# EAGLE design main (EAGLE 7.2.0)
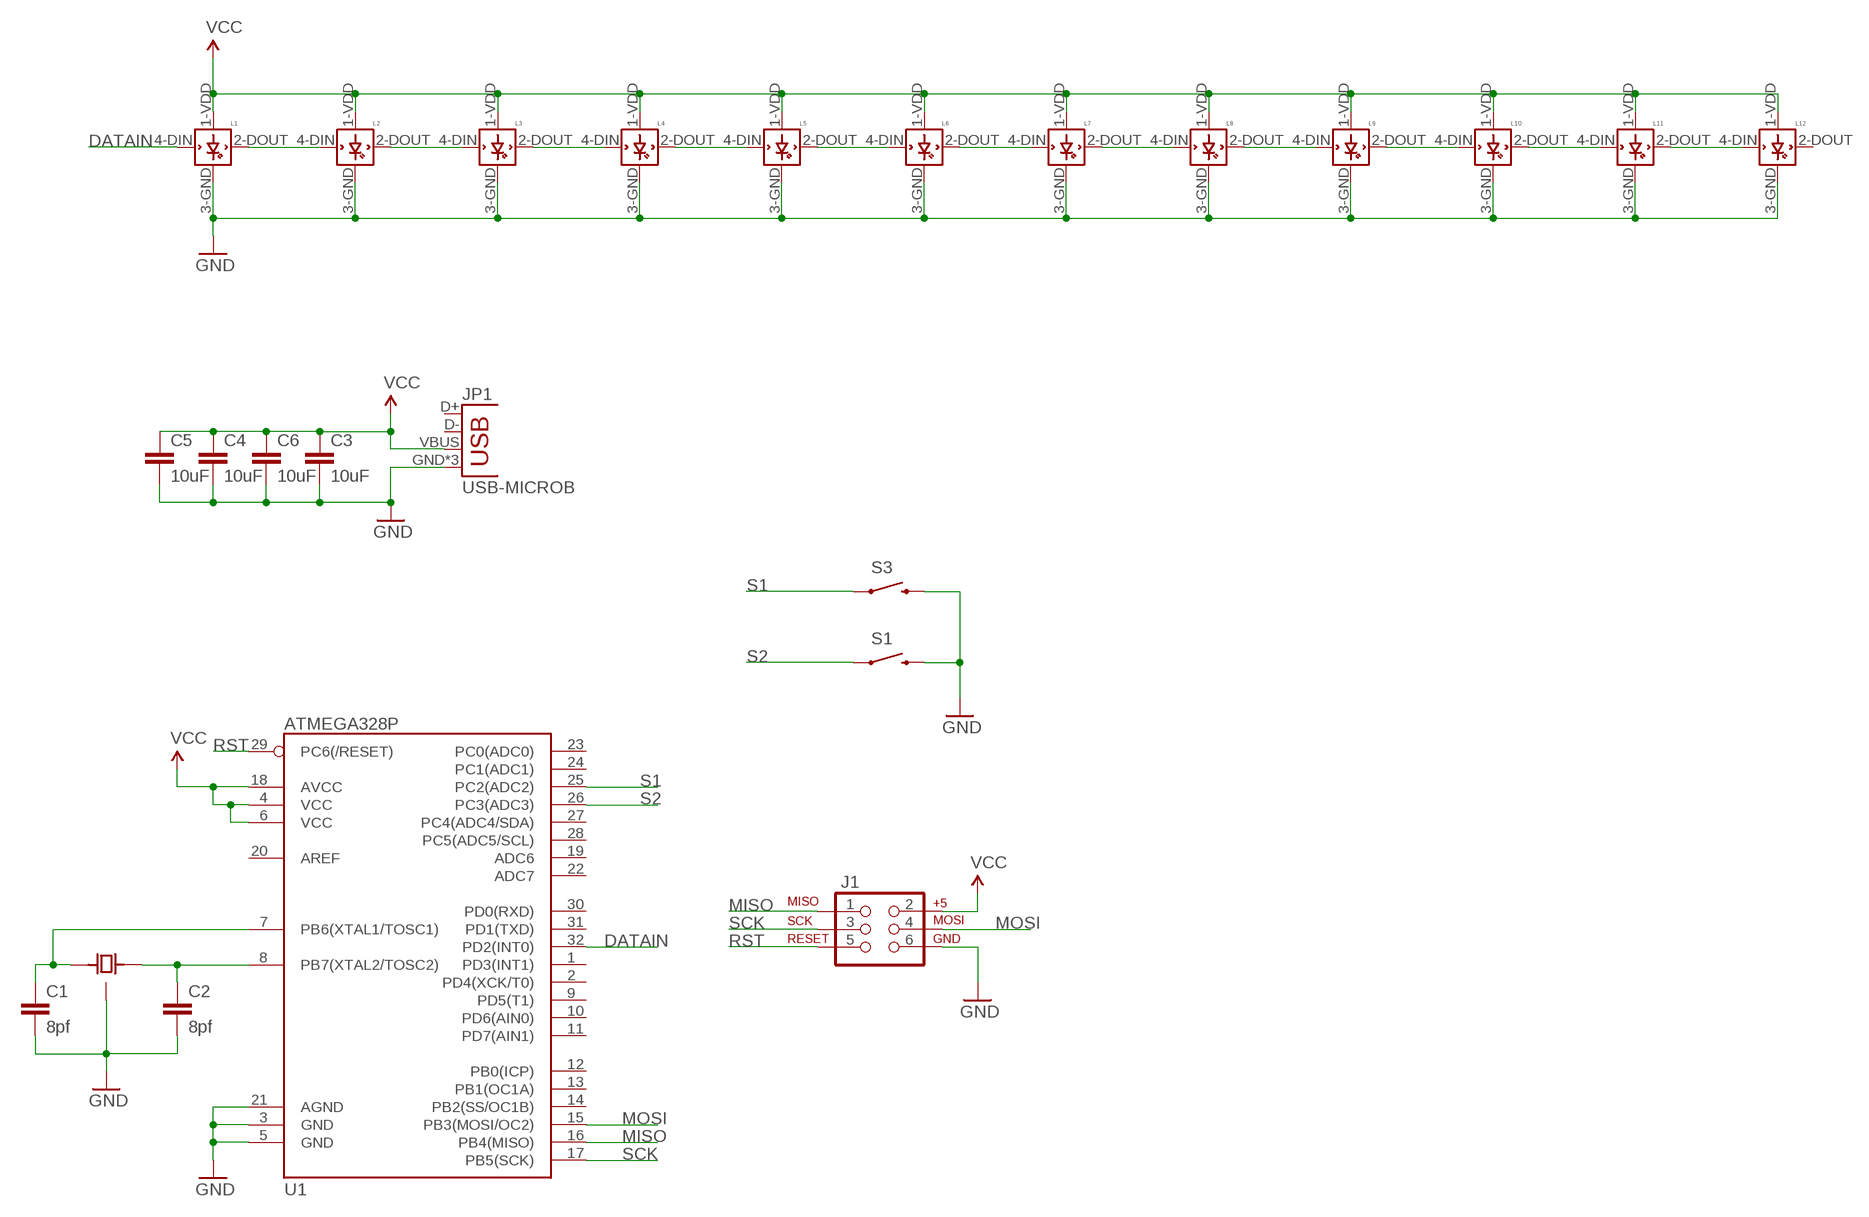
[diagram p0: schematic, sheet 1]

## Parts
C1  8pf  CAP0603-CAP  [0603-CAP]
C2  8pf  CAP0603-CAP  [0603-CAP]
C3  10uF  CAP1206  [1206]
C4  10uF  CAP1206  [1206]
C5  10uF  CAP1206  [1206]
C6  10uF  CAP1206  [1206]
J1  AVR_SPI_PRG_6NS  [2X3-NS]
JP1  USB-MICROB  [USB-MICROB]
L1  WS2812B  [WS2812B]
L2  WS2812B  [WS2812B]
L3  WS2812B  [WS2812B]
L4  WS2812B  [WS2812B]
L5  WS2812B  [WS2812B]
L6  WS2812B  [WS2812B]
L7  WS2812B  [WS2812B]
L8  WS2812B  [WS2812B]
L9  WS2812B  [WS2812B]
L10  WS2812B  [WS2812B]
L11  WS2812B  [WS2812B]
L12  WS2812B  [WS2812B]
S1  SWITCH-MOMENTARY-2SMD-4  [TACTILE_SWITCH_TALL]
S3  SWITCH-MOMENTARY-2SMD-4  [TACTILE_SWITCH_TALL]
U1  ATMEGA328P  ATMEGA328_SMT  [TQFP32-08]
U$1  CRYSTAL_GND  [CRYSTAL-3.2X2.5]

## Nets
DATAIN: L1.4-DIN(DIN) U1.32(PD2(INT0))
GND: C1.2 C2.2 C3.2 C4.2 C5.2 C6.2 J1.6 JP1.GND JP1.MT1(GND) JP1.MT2(GND) L1.3-GND(GND) L2.3-GND(GND) L3.3-GND(GND) L4.3-GND(GND) L5.3-GND(GND) L6.3-GND(GND) L7.3-GND(GND) L8.3-GND(GND) L9.3-GND(GND) L10.3-GND(GND) L11.3-GND(GND) L12.3-GND(GND) S1.B2 S3.B2 U1.3(GND) U1.5(GND) U1.21(AGND) U$1.GND1(GND) U$1.GND2(GND)
MISO: J1.1 U1.16(PB4(MISO))
MOSI: J1.4 U1.15(PB3(MOSI/OC2))
N$1: C2.1 U1.8(PB7(XTAL2/TOSC2)) U$1.2
N$2: C1.1 U1.7(PB6(XTAL1/TOSC1)) U$1.1
N$3: L1.2-DOUT(DOUT) L2.4-DIN(DIN)
N$4: L2.2-DOUT(DOUT) L3.4-DIN(DIN)
N$5: L3.2-DOUT(DOUT) L4.4-DIN(DIN)
N$6: L4.2-DOUT(DOUT) L5.4-DIN(DIN)
N$7: L5.2-DOUT(DOUT) L6.4-DIN(DIN)
N$8: L6.2-DOUT(DOUT) L7.4-DIN(DIN)
N$9: L7.2-DOUT(DOUT) L8.4-DIN(DIN)
N$10: L8.2-DOUT(DOUT) L9.4-DIN(DIN)
N$11: L9.2-DOUT(DOUT) L10.4-DIN(DIN)
N$12: L10.2-DOUT(DOUT) L11.4-DIN(DIN)
N$13: L11.2-DOUT(DOUT) L12.4-DIN(DIN)
RST: J1.5 U1.29(PC6(/RESET))
S1: S3.A2 U1.25(PC2(ADC2))
S2: S1.A2 U1.26(PC3(ADC3))
SCK: J1.3 U1.17(PB5(SCK))
VCC: C3.1 C4.1 C5.1 C6.1 J1.2 JP1.VBUS L1.1-VDD(VDD) L2.1-VDD(VDD) L3.1-VDD(VDD) L4.1-VDD(VDD) L5.1-VDD(VDD) L6.1-VDD(VDD) L7.1-VDD(VDD) L8.1-VDD(VDD) L9.1-VDD(VDD) L10.1-VDD(VDD) L11.1-VDD(VDD) L12.1-VDD(VDD) U1.4(VCC) U1.6(VCC) U1.18(AVCC)
Unconnected: JP1.D+ JP1.D- L12.2-DOUT(DOUT) U1.1(PD3(INT1)) U1.2(PD4(XCK/T0)) U1.9(PD5(T1)) U1.10(PD6(AIN0)) U1.11(PD7(AIN1)) U1.12(PB0(ICP)) U1.13(PB1(OC1A)) U1.14(PB2(SS/OC1B)) U1.19(ADC6) U1.20(AREF) U1.22(ADC7) U1.23(PC0(ADC0)) U1.24(PC1(ADC1)) U1.27(PC4(ADC4/SDA)) U1.28(PC5(ADC5/SCL)) U1.30(PD0(RXD)) U1.31(PD1(TXD))

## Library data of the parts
C1-C6 = SparkFun-Passives:CAP: Capacitor
J1 = SparkFun-Connectors:AVR_SPI_PRG_6: AVR ISP 6 Pin This is the reduced ISP connector for AVR programming. Common on Arduino. This footprint will take up less PCB space and can be used with a 10-pin to 6-pin adapter such as SKU: BOB-08508 **Special note about "TEST_POINT" package. The stop mask is on the top side, so if you want your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
JP1 = SparkFun-Connectors:USB: USB Connectors USB-B-PTH is fully proven SKU : PRT-00139/CONN-08278 USB-miniB is fully proven SKU : PRT-00587 USB-A-PCB is untested. USB-A-H is throughly reviewed, but untested. Spark Fun Electronics SKU : PRT-00437 USB-B-SMT is throughly reviewed, but untested. Needs silkscreen touching up.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; PROD_ID: CONN-09505
L1-L12 = adafruit:WS2812B
S1 S3 = SparkFun-Electromechanical:SWITCH-MOMENTARY-2: Various NO switches- pushbuttons, reed, etc; PROD_ID: SWCH-11966
U1 = SparkFun-DigitalIC:ATMEGA328_SMT: 32-Pin Atmega328 part Commonly used on Arduino compatible boards Available in QFP and QFN packages TQFP is IC-09069 QFN is non-stock; PROD_ID: IC-09069
U$1 = Custom_old:CRYSTAL_GND

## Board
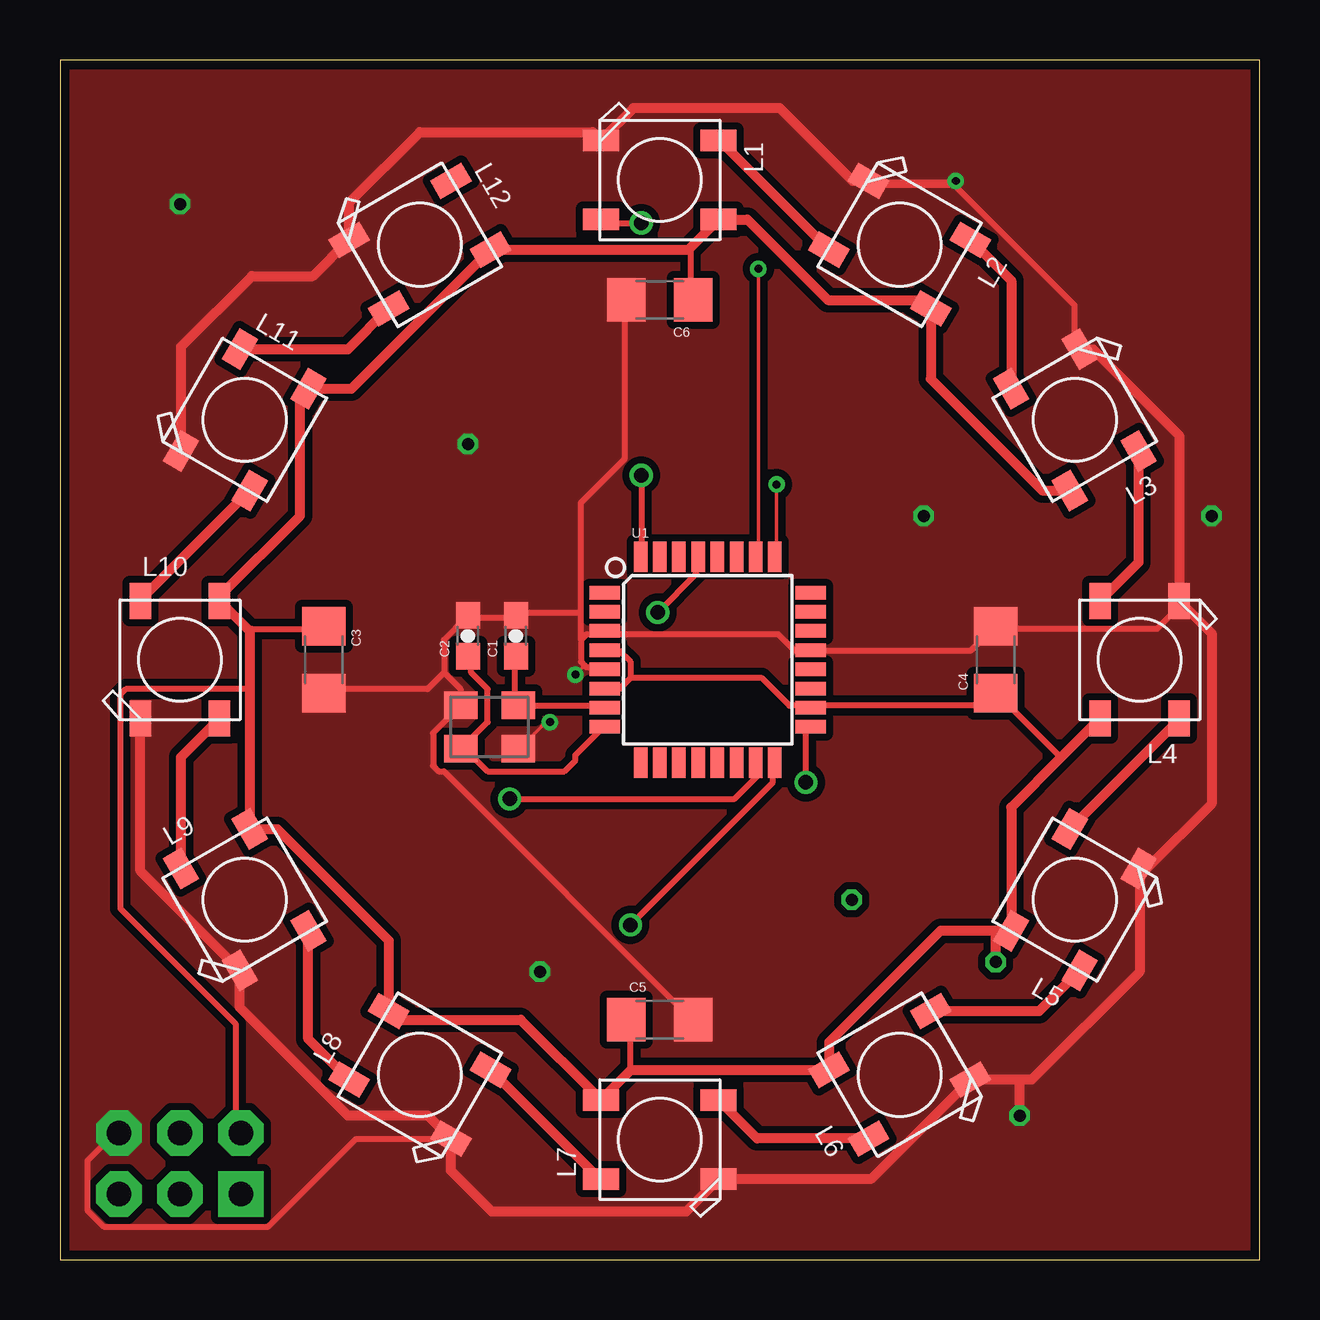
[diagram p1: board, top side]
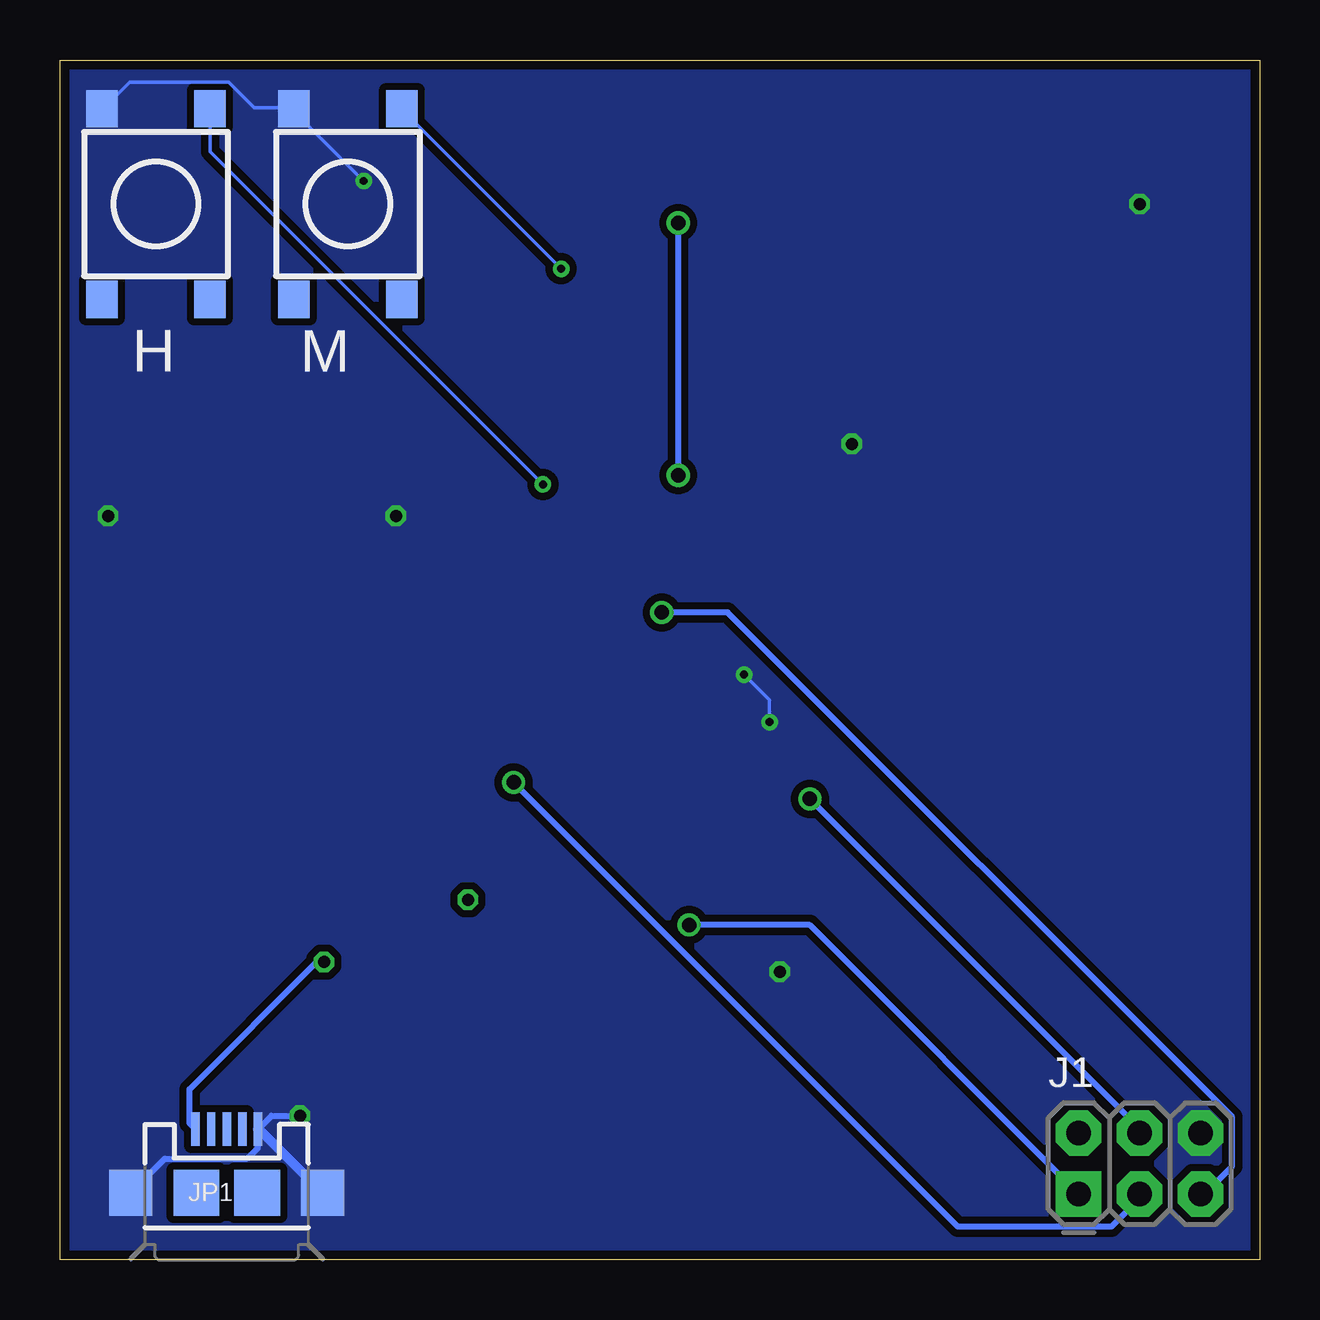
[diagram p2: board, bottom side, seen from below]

Size 50 x 50 mm. Coordinates in mm from the lower left corner, seen from the top.
Outline: 0,0 50,0 50,50 0,50 0,0
Copper layers (1*16): Top 0.0356mm / dielectric 1.5011mm / Bottom 0.0356mm
Design rules "patrick": minimum track width 6mil, minimum drill 13mil, track to track 6mil, track to pad 6mil, pad to pad 6mil, via to via 6mil, smd to smd 6mil, copper to edge 15mil, drill to drill 6mil, minimum pad ring 7mil, minimum via ring 7mil, stop-mask expansion 3mil, vias tented up to drill 30mil, thermal gap 10mil

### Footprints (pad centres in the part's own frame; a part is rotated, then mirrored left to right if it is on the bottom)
0603-CAP = smd 1.1 x 1: 1 -0.85,0; 2 0.85,0
1206 = smd 1.6 x 1.8: 1 -1.4,0; 2 1.4,0
2X3-NS = drill 1.016 pad 1.88 square: 1 -2.54,-1.27 | drill 1.016 pad 1.88 octagon: 2 -2.54,1.27; 3 0,-1.27; 4 0,1.27; 5 2.54,-1.27; 6 2.54,1.27
USB-MICROB = smd 0.35 x 1.4: D+ 0,2.65; D- -0.65,2.65; GND 1.3,2.65; ID 0.65,2.65; VBUS -1.3,2.65 | smd 1.8 x 1.9: MT1 -4,0; MT2 4,0 | smd 1.9 x 1.9: P$1 -1.27,0; P$2 1.27,0
WS2812B = smd 1.5 x 0.9: 1-VDD 2.45,-1.65; 2-DOUT 2.45,1.65; 3-GND -2.45,1.65; 4-DIN -2.45,-1.65
TACTILE_SWITCH_TALL = smd 1.55 x 1.3: A1 -3.975,-2.25; A2 3.975,-2.25; B1 -3.975,2.25; B2 3.975,2.25
TQFP32-08 = smd 1.27 x 0.559: 1 -4.293,2.8; 2 -4.293,2; 3 -4.293,1.2; 4 -4.293,0.4; 5 -4.293,-0.4; 6 -4.293,-1.2; 7 -4.293,-2; 8 -4.293,-2.8; 17 4.293,-2.8; 18 4.293,-2; 19 4.293,-1.2; 20 4.293,-0.4; 21 4.293,0.4; 22 4.293,1.2; 23 4.293,2; 24 4.293,2.8 | smd 0.559 x 1.27: 9 -2.8,-4.293; 10 -2,-4.293; 11 -1.2,-4.293; 12 -0.4,-4.293; 13 0.4,-4.293; 14 1.2,-4.293; 15 2,-4.293; 16 2.8,-4.293; 25 2.8,4.293; 26 2,4.293; 27 1.2,4.293; 28 0.4,4.293; 29 -0.4,4.293; 30 -1.2,4.293; 31 -2,4.293; 32 -2.8,4.293
CRYSTAL-3.2X2.5 = smd 1.4 x 1.15: 1 -0.1,-0.1; 2 2.3,1.7; GND1 -0.1,1.7; GND2 2.3,-0.1

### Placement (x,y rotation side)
C1  19,26 90 top
C2  17,26 90 top
C3  11,25 270 top
C4  39,25 90 top
C5  25,10 0 top
C6  25,40 180 top
J1  5,4 0 bottom
JP1  43.05,2.78 0 bottom
L1  25,45 0 top
L2  35,42.3 330 top
L3  42.3,35 300 top
L4  45,25 270 top
L5  42.3,15 240 top
L6  35,7.7 210 top
L7  25,5 180 top
L8  15,7.7 150 top
L9  7.7,15 120 top
L10  5,25 90 top
L11  7.7,35 60 top
L12  15,42.3 30 top
S1  38,44 90 bottom
S3  46,44 90 bottom
U1  27,25 0 top
U$1  19,23 180 top

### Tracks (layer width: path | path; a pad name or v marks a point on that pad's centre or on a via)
DATAIN  (via drill 0.61)
  Top 0.254: v24.23,32.69 24.23,29.49 U1.32 | v24.23,43.2 22.63,43.2 L1.4-DIN
  Bottom 0.254: v24.23,43.2 v24.23,32.69
GND  (via drill 0.33, 0.5)
  Top 0.152: v20.42,22.4 20.27,22.4 19.2,21.34 U$1.GND1 | 21.87,24.77 v21.49,24.38 | v37.34,44.96 33.83,44.96 L2.3-GND
  Top 0.254: 21.72,25.83 21.72,24.92 21.87,24.77 21.95,24.69 22.63,24.69 U1.5 | 21.72,25.83 21.95,26.06 22.63,26.06 U1.3 22.86,26.06 29.95,26.06 30.63,25.38 31.09,25.38 U1.21 31.32,25.38 37.95,25.38 38.86,26.29 C4.2 39.09,26.29 45.72,26.29 46.63,27.2 L4.3-GND | 21.72,25.83 21.72,26.98 | 21.72,26.98 21.72,31.55 23.55,33.38 23.55,39.78 C6.2 | 16,24.46 16.69,23.77 16.69,23.32 U$1.GND2 16.69,23.09 15.54,21.95 15.54,20.57 15.77,20.34 16,20.34 26.29,10.06 C5.2 | 16,24.46 16,25.83 16.92,26.75 C2.2 17.14,26.75 18.97,26.75 C1.2 19.2,26.98 21.72,26.98 | 16,24.46 15.32,23.77 11.2,23.77 C3.2 | L3.3-GND 42.29,37.95 42.29,39.78 37.26,44.81 33.83,44.81 L2.3-GND | L8.3-GND 16.23,5.03 12.34,5.03 8.69,1.37 1.83,1.37 1.14,2.06 1.14,4.12 2.29,5.26 J1.6
  Top 0.406: L11.3-GND 5.05,38.05 8,41 10.55,41 L12.3-GND 12.05,44.05 15,47 22.2,47 L1.3-GND 23.9,48 30,48 33.05,44.95 L2.3-GND | L3.3-GND 43.05,37.95 46.65,34.35 L4.3-GND 48,26.1 48,19 45.3,16.3 L5.3-GND 45,16.25 45,12 40.5,7.5 40,7.5 | 40,7.5 L6.3-GND 33.8,3.35 L7.3-GND 26.1,2 18,2 16.3,3.7 L8.3-GND 15.34,6 12,6 7.5,10.5 L9.3-GND 3.35,16.2 L10.3-GND | v40,6 40,7.5
  Bottom 0.152: v20.42,22.4 20.42,23.32 v21.49,24.38 | S3.B2 48.16,48.01 47.09,49.07 42.98,49.07 41.91,48.01 40.39,48.01 S1.B2 40.23,47.85 v37.34,44.96
  Bottom 0.254: JP1.MT1 45.63,4.2 42.2,4.2 41.75,4.65 JP1.GND 41.18,6 v40,6
  Bottom 0.406: JP1.MT2 41.7,5.43 JP1.GND
  other vias: 5,44 17,34 36,31 48,31 20,12
  pour Bottom (isolate 0.305, no thermals): 0,50 0,0 50,0 50,50
  pour Top (isolate 0.305, no thermals): 0,50 50,50 50,0 0,0
MISO  (via drill 0.61)
  Top 0.254: v23.77,13.95 29.72,19.89 29.72,20.57 U1.16
  Bottom 0.254: v23.77,13.95 18.75,13.95 7.54,2.74 J1.1
MOSI  (via drill 0.61)
  Top 0.254: v18.75,19.2 28.12,19.2 29.03,20.12 29.03,20.57 U1.15
  Bottom 0.254: v18.75,19.2 5.03,5.49 J1.4
N$1
  Top 0.254: C2.1 17.14,25.15 17.14,24.46 17.83,23.77 17.83,22.4 16.92,21.49 U$1.2 16.92,21.26 17.83,20.34 21.03,20.34 21.49,20.8 21.49,21.03 22.63,22.17 U1.8
N$2
  Top 0.254: C1.1 18.97,25.15 18.97,23.32 U$1.1 19.2,23.09 22.63,23.09 U1.7
N$3
  Top 0.406: L1.2-DOUT 27.5,46.65 L2.4-DIN
N$4
  Top 0.406: L2.2-DOUT 39.65,40.8 L3.4-DIN
N$5
  Top 0.406: L3.2-DOUT 44.95,29.05 L4.4-DIN
N$6
  Top 0.406: L4.2-DOUT 46.65,22.5 L5.4-DIN
N$7
  Top 0.406: L5.2-DOUT 40.8,10.35 L6.4-DIN
N$8
  Top 0.406: L6.2-DOUT 29.05,5.05 L7.4-DIN
N$9
  Top 0.406: L7.2-DOUT 22.5,3.35 L8.4-DIN
N$10
  Top 0.406: L8.2-DOUT 10.35,9.2 L9.4-DIN
N$11
  Top 0.406: L9.2-DOUT 5.05,20.95 L10.4-DIN
N$12
  Top 0.406: L10.2-DOUT 3.35,27.5 L11.4-DIN
N$13
  Top 0.406: L11.2-DOUT 12,37.95 L12.4-DIN
N$17  (via drill 0.5)
  other vias: 33,15
RST  (via drill 0.61)
  Top 0.254: v24.92,26.98 26.52,28.57 26.52,29.26 U1.29
  Bottom 0.254: v24.92,26.98 22.17,26.98 1.14,5.94 1.14,3.89 2.29,2.74 J1.5
S1  (via drill 0.33)
  Top 0.152: v29.87,32.31 29.87,29.41 U1.25
  Bottom 0.152: v29.87,32.31 43.74,46.18 43.74,47.85 S3.A2
S2  (via drill 0.33)
  Top 0.152: v29.11,41.3 29.11,29.41 U1.26
  Bottom 0.152: v29.11,41.3 35.66,47.85 S1.A2
SCK  (via drill 0.61)
  Top 0.254: v31.09,19.89 31.09,22.17 U1.17
  Bottom 0.254: v31.09,19.89 12.57,1.37 6.17,1.37 5.03,2.52 J1.3
VCC  (via drill 0.5)
  Top 0.254: 23.77,24.23 23.32,23.77 22.86,23.77 U1.6 | 23.77,24.23 23.77,24.92 23.32,25.38 22.86,25.38 U1.4 | 23.77,24.23 29.26,24.23 30.4,23.09 31.09,23.09 U1.18 31.32,23.09 38.41,23.09 38.86,23.55 C4.1 39.09,23.55 41.72,20.92 | C5.1 23.77,9.83 23.77,8 23.8,7.9 | C3.1 10.97,26.29 8,26.29 7.9,26.2 | C6.1 26.29,40.01 26.29,42.06 26.2,42.1 | 7.9,23.77 2.74,23.77 2.52,23.55 2.52,14.63 7.32,9.83 7.32,5.49 J1.2
  Top 0.406: L3.1-VDD 40.95,32.05 36.3,36.7 L2.1-VDD 35.94,40 32,40 28.65,43.35 L1.1-VDD 26.2,42.1 L12.1-VDD 12.15,36.3 L11.1-VDD 10,35.94 10,31 6.65,27.65 L10.1-VDD 7.9,26.2 7.9,23.77 L9.1-VDD 9.05,17.95 13.7,13.3 L8.1-VDD 14.06,10 19.2,10 L7.1-VDD 23.8,7.9 L6.1-VDD 32.05,9.05 36.7,13.7 39,13.7 | L4.1-VDD 41.72,20.92 39.65,18.85 L5.1-VDD 39,13.7 | v39,12.4 39,13.7
  Bottom 0.254: JP1.VBUS 44.6,5.68 44.6,7.1 39.3,12.4 v39,12.4

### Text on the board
bPlace: M | H

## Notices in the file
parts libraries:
SparkFun-DigitalIC: Licensing: Creative Commons ShareAlike 4.0 International - https://creativecommons.org/licenses/by-sa/4.0
